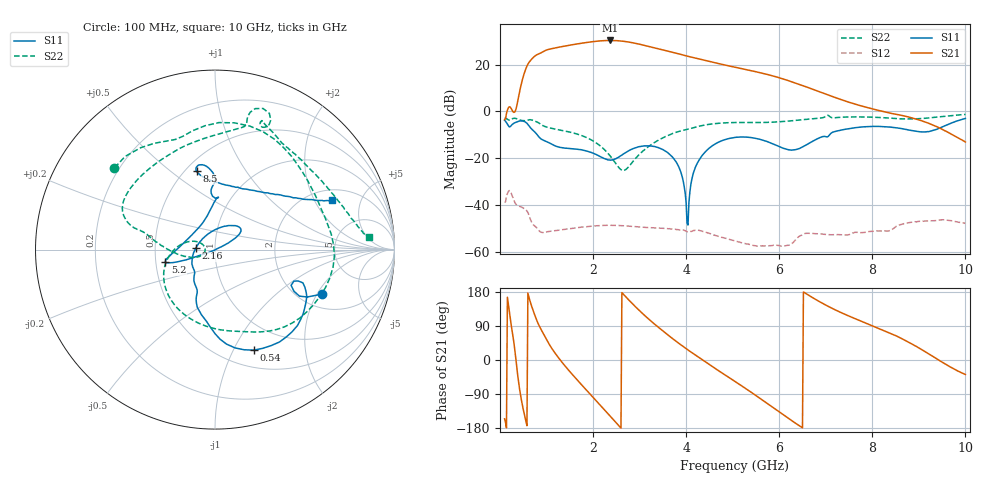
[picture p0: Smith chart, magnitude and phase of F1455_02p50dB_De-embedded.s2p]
! Integrated Device Technology
! Corporate Headquarters
! 6024 Silver Creek Valley Road
! San Jose, CA 95138  USA
! Phone:  1-408-284-8200
! Toll Free:  1-800-223-1366
! Webpage:  http://www.idt.com/
! Timing and RF Division
! 515 Groton Road, Suite 102
! Westford, MA 01886-6024
! Device:  F1455
! Description: 6-bit 0.5 dB Transmit Variable Gain Amplifier
! Frequency:  1400.0 -  2300.00 MHz
! Package:  6x6 mm Thin QFN Plastic Package: 28 pin
! State:  5
! Atten State:  2.5 dB
! Voltage:  +5.00 Volts
! Current:  214.720 mA
! Data:  The device was measured on a the F1455 evaluation board which has
!  individual transmission lines to the RF pins.  Data was collected
!  using a calibrated network analyzer.  The evaluation board was
!  de-embedded using a TRL calibration technique.
!  The reference plane is the edge of the package pin.
!  Pin  1 = CSb
!  Pin  2 = DATA
!  Pin  3 = CLK
!  Pin  4 = RSET
!  Pin  5 = GND
!  Pin  6 = RFIN  = Port 1
!  Pin  7 = GND
!  Pin  8 = NC
!  Pin  9 = NC
!  Pin 10 = NC
!  Pin 11 = NC
!  Pin 12 = NC
!  Pin 13 = NC
!  Pin 14 = /STBY
!  Pin 15 = GND
!  Pin 16 = RFOUT  = Port 2
!  Pin 17 = GND
!  Pin 18 = NC
!  Pin 19 = NC
!  Pin 20 = NC
!  Pin 21 = GND
!  Pin 22 = NC
!  Pin 23 = GND
!  Pin 24 = NC
!  Pin 25 = NC
!  Pin 26 = NC
!  Pin 27 = GND
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# GHz S dB R 50
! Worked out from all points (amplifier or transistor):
!   496 points, 100 MHz to 10 GHz, reference 50 ohm
!   highest |S21| = 30.3 dB at 2.36 GHz (marker M1)
!   |S21| within 3 dB of that: 1.237 GHz to 3.289 GHz (2.052 GHz wide, 90.7 % of centre)
!   unconditionally stable (mu >= 1): start of sweep to end of sweep
!   at 1.74 GHz: K = 4.63, MAG = 29.7 dB, |S12| = -49.5 dB
!   at 5.06 GHz: K = 20.51, MAG = 21.0 dB, |S12| = -55.3 dB
!   at 10 GHz: K = 70.53, MAG = -4.1 dB, |S12| = -47.8 dB
!   S11 on the Smith chart (normalised r, x): 100 MHz: 2.58, -2.20; 540 MHz: 0.69, -1.21; 2.16 GHz: 0.81, +0.01; 5.2 GHz: 0.56, -0.08; 8.5 GHz: 0.57, +0.62; 10 GHz: 2.53, +2.80
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0.1  -3.82 -22.7  -3.49 -155.3  -38.94 40.0  -2.83 140.8
0.4  -4.21 -39.2  6.22 -58.2  -40.37 -111.8  -3.45 50.6
0.54  -4.43 -69.0  17.37 -152.3  -41.72 -158.2  -3.96 20.5
0.7  -7.90 -96.8  22.74 134.9  -48.02 152.4  -3.74 -19.2
0.96  -12.52 -116.0  25.90 63.2  -51.67 125.2  -6.39 -72.3
1.14  -14.30 -127.4  26.95 25.9  -51.04 103.5  -7.34 -96.6
1.34  -15.50 -132.7  27.75 -7.0  -50.53 82.0  -8.13 -120.0
1.76  -16.42 -148.4  29.17 -66.2  -49.41 47.7  -10.33 -158.7
1.96  -17.51 -161.4  29.74 -92.9  -49.05 34.1  -12.13 -175.0
2.16  -19.37 176.0  30.16 -119.8  -48.76 21.3  -14.80 169.2
2.36  -20.74 137.2  30.34 -147.1  -48.64 8.9  -18.80 156.8
2.62  -18.65 83.3  30.07 177.8  -48.84 -6.1  -25.12 174.3
2.92  -15.46 52.7  29.08 139.5  -49.24 -20.6  -19.90 -156.9
3.4  -15.44 33.7  26.79 86.7  -49.86 -40.3  -12.34 -177.7
4.04  -48.55 -131.1  23.56 26.5  -51.46 -65.1  -7.57 166.0
5.06  -11.07 -164.9  18.86 -57.5  -55.34 -102.7  -4.72 148.9
5.2  -10.90 -166.1  18.27 -68.8  -56.15 -104.3  -4.70 144.4
5.94  -14.48 172.3  14.77 -131.9  -57.15 -105.3  -4.48 109.1
6.7  -12.95 96.4  9.64 165.8  -52.08 -133.6  -3.20 78.3
8.36  -6.64 103.1  -0.62 71.6  -51.03 171.1  -2.83 62.4
8.5  -6.94 103.2  -1.17 64.4  -49.34 172.8  -3.05 58.5
10  -3.00 22.9  -13.06 -38.2  -47.83 85.8  -1.29 4.6
